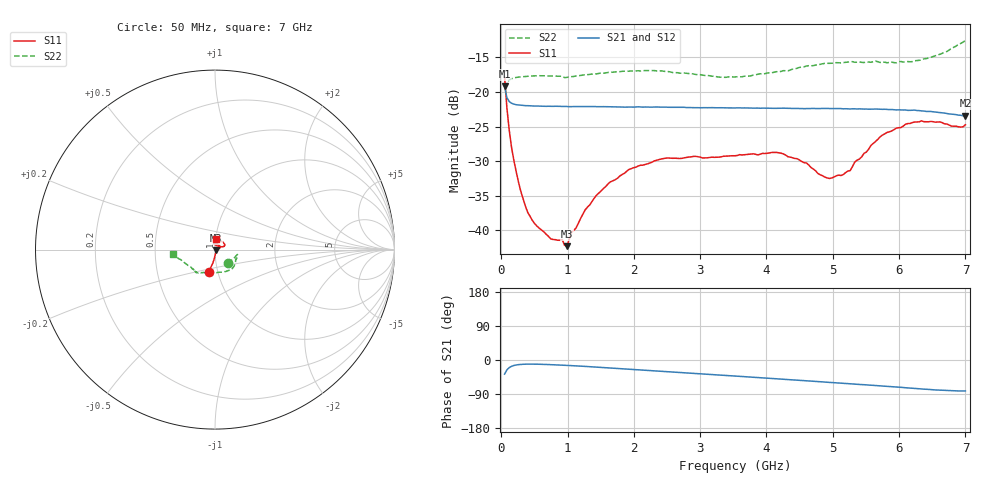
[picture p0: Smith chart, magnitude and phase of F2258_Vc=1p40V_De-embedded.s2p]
! Integrated Device Technology
! Corporate Headquarters
! 6024 Silver Creek Valley Road
! San Jose, CA 95138  USA
! Phone:  1-408-284-8200
! Toll Free:  1-800-223-1366
! Webpage:  http://www.idt.com/
! Timing and RF Division
! 515 Groton Road, Suite 102
! Westford, MA 01886-6024
! Device:  F2258
! Description: Voltage Variable RF Attenuator
! Frequency:  50.0 -  6000.00 MHz
! Package:  3x3 mm Thin QFN Plastic Package: 16 pin
! Ports:  2 RF, 2 DC
!  Pin  1  = NC
!  Pin  2  = NC
!  Pin  3  = RF2  = Port 2
!  Pin  4  = GND
!  Pin  5  = Vdd
!  Pin  6  = NC
!  Pin  7  = VCTRL
!  Pin  8  = NC
!  Pin  9  = GND
!  Pin 10  = RF1  = Port 1
!  Pin 11  = NC
!  Pin 12  = NC
!  Pin 13  = NC
!  Pin 14  = NC
!  Pin 15  = NC
!  Pin 16  = NC
! Vcntrl:  1.400 Volts
! Vdd:  +3.300 Volts
! Current:  1.164 mA
! Data:  The device was measured on a the F2258 evaluation board which has
!  individual transmission lines to the RF pins.  Data was collected
!  using a calibrated network analyzer.  The evaluation board was
!  de-embedded using a TRL calibration technique.
!  The reference plane is the edge of the package pin.
! Misc:  SN 10
!  Action Tracker AT0285
! Date Measured:  2014-12-10
! Date:  2016-01-13  MJV
! Note:
!  Integrated Device Technology supplies this data as a sample of measured
!  data at the package pin for this product.  Your particular data for this
!  product may vary.
!  Data was taken at 25 degrees C.
!  Integrated Device Technology reserves the right to change this data at anytime.
!Freq_(GHz)  S11M_(dB)  S11P_(deg)  S21M_(dB)  S21P_(deg)  S12M_(dB)  S12P_(deg)  S22M_(dB)  S22P_(deg)
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# GHz S dB R 50
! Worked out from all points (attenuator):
!   201 points, 50 MHz to 7 GHz, reference 50 ohm
!   highest |S21| = -19.16 dB at 50 MHz (marker M1); lowest = -23.4 dB at 7 GHz (marker M2)
!   lowest |S11| = -42.3 dB at 988.2 MHz (marker M3), VSWR 1.02, Z = 50.7 - j0.35 ohm
!   |S11| at or under -10 dB: start of sweep to end of sweep
!   |S22| runs from -19.5 to -12.5 dB; largest |S21 - S12| = 0.00049
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0.05  -17.86 -105.8  -19.16 -37.2  -19.15 -37.2  -19.51 -46.9
0.08475  -22.33 -99.2  -20.82 -26.0  -20.79 -25.9  -18.68 -23.8
0.15425  -27.99 -92.5  -21.63 -16.7  -21.58 -16.6  -18.09 -14.6
0.2585  -32.99 -83.9  -21.88 -12.3  -21.85 -12.2  -17.85 -12.2
0.36275  -36.50 -74.5  -21.98 -11.0  -21.97 -11.0  -17.74 -12.8
0.5365  -39.40 -55.1  -22.03 -11.0  -22.04 -11.0  -17.65 -15.3
0.91875  -41.34 -10.6  -22.10 -13.6  -22.11 -13.6  -17.72 -23.9
0.98825  -42.31 -26.7  -22.10 -14.2  -22.12 -14.2  -17.89 -25.3
1.05775  -40.33 -16.1  -22.12 -14.8  -22.09 -14.9  -17.78 -26.6
1.2315  -37.64 -3.2  -22.09 -16.6  -22.10 -16.6  -17.55 -30.2
1.6485  -33.00 8.4  -22.13 -21.1  -22.16 -21.1  -17.16 -38.4
1.9265  -31.21 17.3  -22.17 -24.1  -22.17 -24.1  -16.98 -43.7
2.37825  -29.77 29.1  -22.19 -29.1  -22.21 -29.1  -16.95 -52.8
3.525  -29.23 81.7  -22.32 -42.3  -22.29 -42.3  -17.83 -89.4
4.18525  -28.80 101.6  -22.36 -50.0  -22.36 -50.0  -17.09 -112.8
4.7065  -31.14 90.8  -22.39 -56.1  -22.38 -56.1  -16.18 -123.6
4.94975  -32.52 69.9  -22.41 -59.0  -22.38 -59.1  -15.86 -126.5
5.15825  -31.94 48.6  -22.44 -61.5  -22.40 -61.6  -15.75 -128.5
5.71425  -26.48 19.6  -22.49 -68.3  -22.48 -68.4  -15.73 -133.2
5.85325  -25.77 20.2  -22.55 -70.1  -22.51 -70.2  -15.74 -135.9
6.33975  -24.18 28.0  -22.74 -76.5  -22.75 -76.5  -15.34 -148.2
7  -24.75 83.7  -23.45 -81.7  -23.40 -81.9  -12.55 -173.4
